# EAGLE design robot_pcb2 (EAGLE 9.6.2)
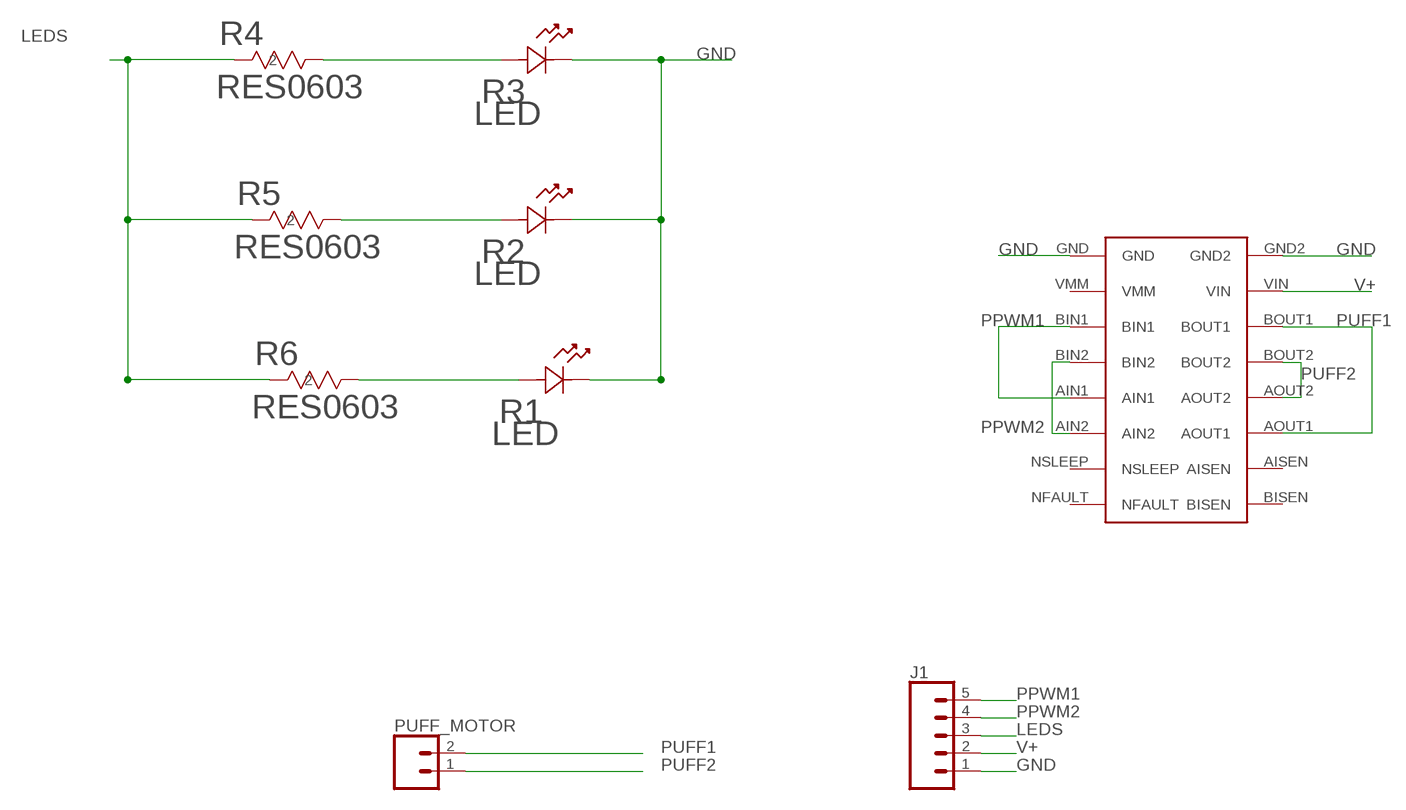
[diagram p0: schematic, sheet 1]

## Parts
J1  CONN_05  [1X05]
PUFF_MOTOR  CONN_02  [CONN_02]
R1  LED  [LED]
R2  LED  [LED]
R3  LED  [LED]
R4  RES0603  [RES0603]
R5  RES0603  [RES0603]
R6  RES0603  [RES0603]
U$2  DRV8833_BREAKOUT  [DRV8833_BREAKOUT]

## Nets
GND: J1.1 R1.1 R2.1 R3.1 U$2.GND U$2.GND2
LEDS: J1.3 R4.2 R5.2 R6.2
N$1: R3.2 R4.1
N$2: R2.2 R5.1
N$3: R1.2 R6.1
PPWM1: J1.5 U$2.AIN1 U$2.BIN1
PPWM2: J1.4 U$2.AIN2 U$2.BIN2
PUFF1: PUFF_MOTOR.2 U$2.AOUT1 U$2.BOUT1
PUFF2: PUFF_MOTOR.1 U$2.AOUT2 U$2.BOUT2
V+: J1.2 U$2.VIN
Unconnected: U$2.AISEN U$2.BISEN U$2.NFAULT U$2.NSLEEP U$2.VMM

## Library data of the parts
J1 = maciver_robot_lib:CONN_05: Multi connection point. Often used as Generic Header-pin footprint for 0.1 inch spaced/style header connections On any of the 0.1 inch spaced packages, you can populate with these: Break Away Headers - Straight (PRT-00116) Break Away Male Headers - Right Angle (PRT-00553) Female Headers (PRT-00115)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
PUFF_MOTOR = maciver_robot_lib:CONN_02: Multi connection point. Often used as Generic Header-pin footprint for 0.1 inch spaced/style header connections
R1-R3 = maciver_robot_lib:LED; BUILT_BY: EMA_Matt; COPYRIGHT: Copyright (C) 2018 Accelerated Designs. All rights reserved; MANUFACTURER_PART_NUMBER: SML-512UWT86; SOURCELIBRARY: Rohm_2019-09-23; VENDOR: ROHM Semiconductor
R4-R6 = maciver_robot_lib:RES0603; BUILT_BY: EMA_UL_Team; MANUFACTURER_PART_NUMBER: ERJ-3GEYJ103V; SOURCELIBRARY: Panasonic_2010-01-01_Res5; VENDOR: Panasonic
U$2 = maciver_robot_lib:DRV8833_BREAKOUT

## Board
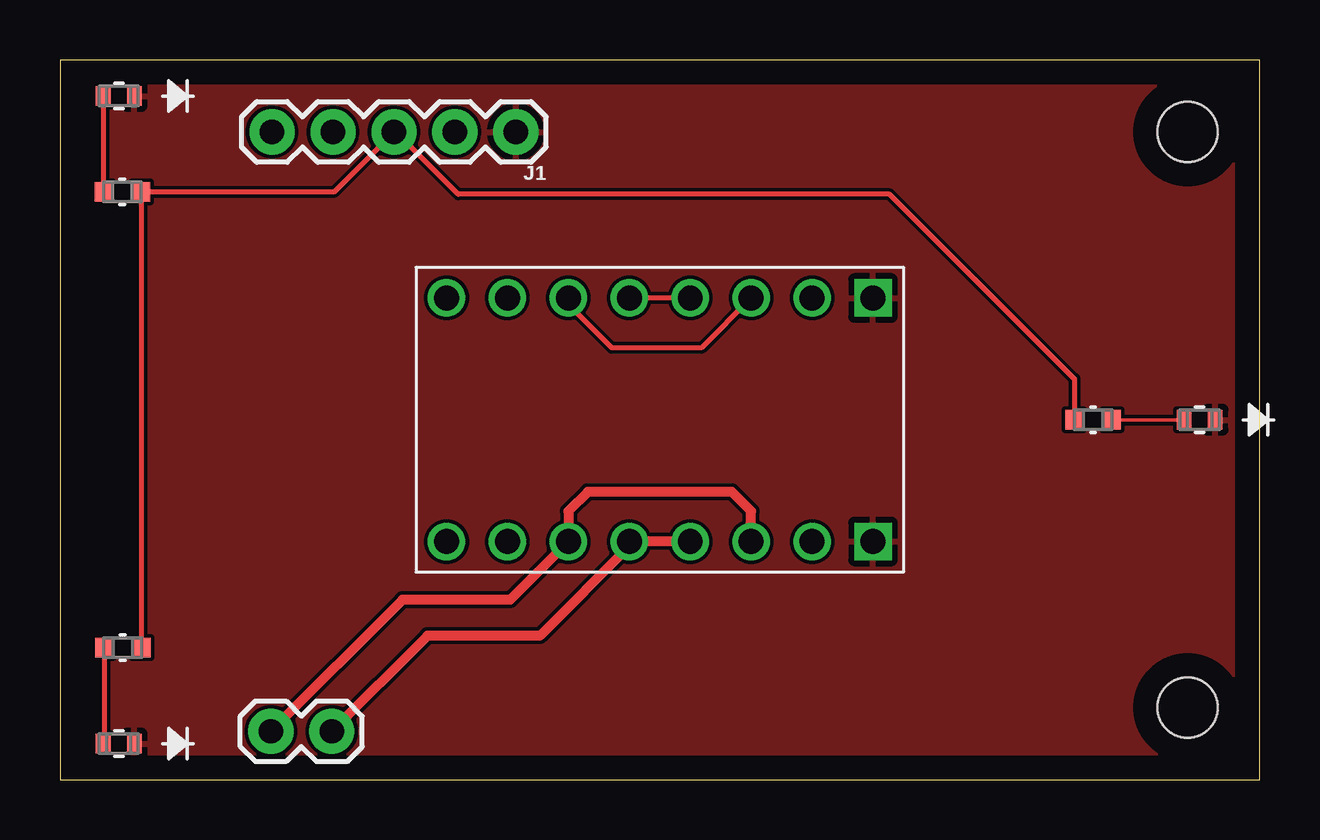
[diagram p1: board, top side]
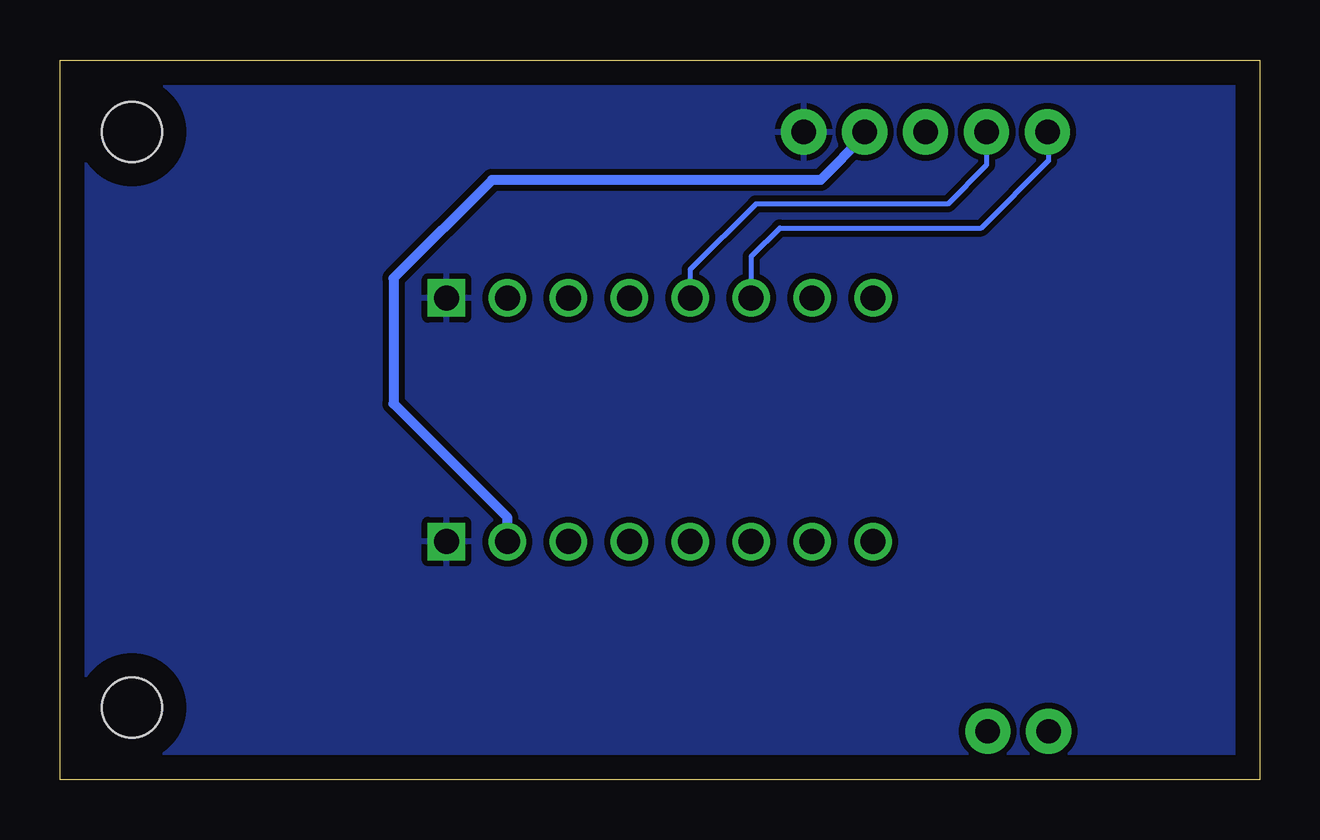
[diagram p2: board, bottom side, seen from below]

Size 50 x 30 mm. Coordinates in mm from the lower left corner, seen from the top.
Outline: 0,0 50,0 50,30 0,30 0,0
Copper layers (1*16): Top 0.035mm / dielectric 1.5mm / Bottom 0.035mm
Design rules "default": minimum track width 6mil, minimum drill 0.35mm, track to track 6mil, track to pad 6mil, pad to pad 6mil, via to via 6mil, smd to smd 6mil, copper to edge 40mil, drill to drill 6mil, minimum pad ring 10mil, minimum via ring 8mil, stop-mask expansion 4mil, vias tented up to drill 0mil, thermal gap 10mil
Holes 2.5 mm at 47,27 47,3

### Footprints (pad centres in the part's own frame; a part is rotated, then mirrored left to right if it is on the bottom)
1X05 = drill 1.016 pad 1.88: 1 0,0; 2 2.54,0; 3 5.08,0; 4 7.62,0; 5 10.16,0
CONN_02 = drill 1.016 pad 1.88: 1 0,0; 2 2.54,0
LED = smd 0.61 x 0.813: 1 -0.648,0; 2 0.648,0
RES0603 = smd 0.756 x 0.8: 1 -0.778,0; 2 0.778,0
DRV8833_BREAKOUT = drill 1.04: AIN1 -5.08,-3.81; AIN2 -5.08,-1.27; AISEN 5.08,-6.35; AOUT1 5.08,-3.81; AOUT2 5.08,-1.27; BIN1 -5.08,3.81; BIN2 -5.08,1.27; BISEN 5.08,-8.89; BOUT1 5.08,3.81; BOUT2 5.08,1.27; NFAULT -5.08,-8.89; NSLEEP -5.08,-6.35; VIN 5.08,6.35; VMM -5.08,6.35 | drill 1.04 square: GND -5.08,8.89; GND2 5.08,8.89

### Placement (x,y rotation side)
J1  19,27 180 top
PUFF_MOTOR  11.33,2.01 180 top
R1  2.45,1.5 180 top
R2  47.5,15 180 top
R3  2.45,28.5 180 top
R4  2.6,24.5 0 top
R5  43.06,15 180 top
R6  2.62,5.5 0 top
U$2  25,15 270 top

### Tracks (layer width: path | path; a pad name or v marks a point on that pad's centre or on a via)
GND
  pour Top: 0,30 50,30 50,0 0,0
  pour Top (isolate 12): 0,30 50,30 50,0 0,0
  pour Bottom (isolate 0.254): 0,30 0,0 50,0 50,30
LEDS
  Top 0.203: R5.2 42.28,16.7 34.58,24.4 16.6,24.4 14,27 J1.3 11.42,24.5 R4.2 3.38,5.52 R6.2
N$1
  Top 0.203: R4.1 1.82,28.48 R3.2
N$2
  Top 0.152: R5.1 R2.2
N$3
  Top 0.203: R6.1 1.84,1.54 R1.2
PPWM1
  Top 0.203: U$2.BIN1 26.73,18 23,18 21.19,19.81 U$2.AIN1
  Bottom 0.203: U$2.AIN1 21.19,21.81 20,23 11.6,23 8.8,25.8 8.8,26.96 J1.5
PPWM2
  Top 0.203: U$2.BIN2 U$2.AIN2
  Bottom 0.203: U$2.AIN2 23.73,21.27 21,24 13,24 11.38,25.62 J1.4
PUFF1
  Top 0.406: U$2.BOUT1 28.81,11.19 28,12 22,12 21.19,11.19 U$2.AOUT1 18.77,7.5 14.28,7.5 PUFF_MOTOR.2
PUFF2
  Top 0.406: PUFF_MOTOR.1 15.32,6 20,6 23.73,9.73 U$2.AOUT2 U$2.BOUT2
V+
  Bottom 0.406: U$2.VIN 31.35,10.92 36.1,15.67 36.1,20.9 32,25 18.3,25 16.46,26.84 J1.2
